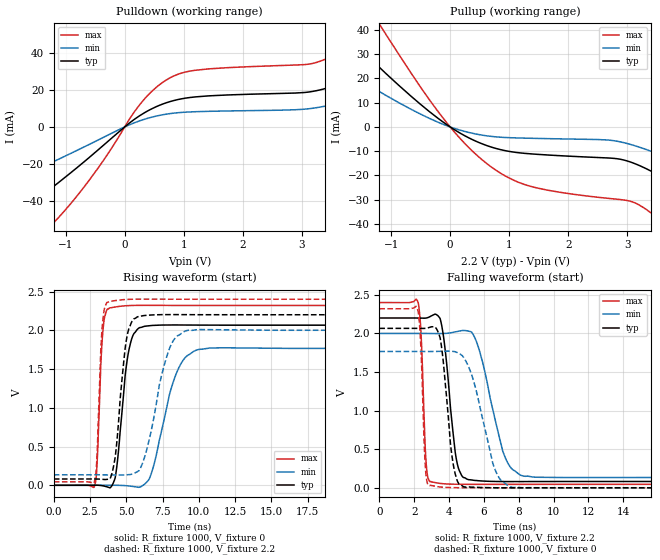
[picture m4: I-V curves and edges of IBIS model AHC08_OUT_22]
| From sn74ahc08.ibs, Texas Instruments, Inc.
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[Model]   AHC08_OUT_22
Model_type  Output
Vref =   0
Rref =   1000
Cref =   50p
Vmeas =   1.1
| variable   typ   min   max
C_comp   3.23pF   2.16pF   4.32pF
| C_pullup   3.15pF   2.16pF   3.84pF
| C_pulldown   3.32pF   2.17pF   4.32pF
[Temperature Range]   40   100   -40
| Ambient temperature   25   85   -40
[Voltage range]   2.2   2   2.4
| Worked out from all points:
|   slope of the pulldown table from 0 to 0.33 V, typ, clamps not added: 43.7 ohm
|   slope of the pullup table from 0 to 0.33 V, typ, clamps not added: 70.6 ohm
|   rising waveform, R_fixture 1000, V_fixture 0: 20-80 % time 645ps typ, 1.37ns min, 302ps max; typ from 0 V to 2.07 V
|   falling waveform, R_fixture 1000, V_fixture 2.2: 20-80 % time 549ps typ, 1.12ns min, 228ps max; typ from 2.2 V to 0.081 V
|   rising waveform, R_fixture 1000, V_fixture 2.2: 20-80 % time 608ps typ, 1.26ns min, 286ps max; typ from 0.081 V to 2.2 V
|   falling waveform, R_fixture 1000, V_fixture 0: 20-80 % time 507ps typ, 1.1ns min, 220ps max; typ from 2.07 V to 0 V
[Pulldown]
| AHC08_OUT_22
|   Voltage   I(typ)   I(min)   I(max)
-5.5V     -129.7mA   -81.96mA   -163.3mA
-3.52V    -85.27mA   -52.66mA   -112.8mA
-2.06V    -52.71mA   -31.41mA   -76.14mA
-1.305V   -34.6mA    -20.22mA   -55.05mA
-620mV    -17.01mA   -9.739mA   -29.56mA
255mV     6.077mA    3.299mA    12.04mA
700mV     12.99mA    6.867mA    25.22mA
3.18V     19.13mA    10.06mA    34.23mA
4.255V    31.65mA    18.76mA    53.81mA
5.495V    55.86mA    35.18mA    90.99mA
6.65V     83.86mA    53.91mA    133.1mA
11V       219.4mA    135.9mA    343.2mA
[Pullup]
| AHC08_OUT_22
|   Voltage   I(typ)   I(min)   I(max)
-5.5V     148.2mA    89.86mA    250.9mA
-2.925V   68.89mA    42.38mA    115.6mA
-1.835V   39.98mA    24.23mA    67.91mA
-1.28V    26.5mA     15.78mA    45.63mA
-75mV     1.249mA    669.7uA    2.265mA
735mV     -8.599mA   -4.003mA   -17.2mA
1.465V    -11.29mA   -4.739mA   -25.17mA
3.09V     -14.81mA   -7.487mA   -30.98mA
3.665V    -21.78mA   -12.51mA   -40.65mA
4.85V     -41.88mA   -25.99mA   -67.56mA
5.975V    -64.03mA   -40.67mA   -94.77mA
11V       -175.9mA   -114.5mA   -224.3mA
[Ramp]
| AHC08_OUT_22
| variable   typ   min   max
dV/dt_r   1.26/7.22E-10   1.08/1.50E-09   1.41/3.33E-10
dV/dt_f   1.30/5.74E-10   1.14/1.16E-09   1.44/2.42E-10
R_load = 1000
[Rising Waveform]
| AHC08_OUT_22
R_fixture =   1000
C_fixture =   0
L_fixture =   0
V_fixture =   0
V_fixture_min = 0
V_fixture_max = 0
|   Time   V(typ)   V(min)   V(max)
0s        158.4pV    433.8pV    54.03pV
2.815ns   921.6uV    339uV      -4.923mV
3.375ns   -6.447mV   471.4uV    1.971V
3.88ns    -33.16mV   455.6uV    2.29V
4.305ns   186.6mV    50.2uV     2.302V
5.19ns    1.758V     -9.166mV   2.318V
6.24ns    2.051V     11.07mV    2.322V
8.45ns    2.068V     1.445V     2.32V
9.995ns   2.067V     1.753V     2.32V
50ns      2.066V     1.766V     2.32V
[Falling Waveform]
| AHC08_OUT_22
R_fixture =   1000
C_fixture =   0
L_fixture =   0
V_fixture =   2.2
V_fixture_min = 2
V_fixture_max = 2.4
|   Time   V(typ)   V(min)   V(max)
0s        2.2V       2V         2.4V
2.24ns    2.199V     2V         2.392V
2.68ns    2.199V     2V         349.2mV
2.915ns   2.218V     1.999V     78.02mV
3.53ns    2.159V     1.998V     55.22mV
4.41ns    387.2mV    2.022V     45.51mV
5.125ns   104.6mV    2.03V      44.03mV
7.16ns    80.3mV     429.3mV    43.92mV
8.28ns    80.22mV    150.6mV    44.1mV
50ns      81.22mV    134.8mV    44.2mV
[Rising Waveform]
| AHC08_OUT_22
R_fixture =   1000
C_fixture =   0
L_fixture =   0
V_fixture =   2.2
V_fixture_min = 2
V_fixture_max = 2.4
|   Time   V(typ)   V(min)   V(max)
0s        81.22mV    134.8mV    44.2mV
2.79ns    81.49mV    135.2mV    41.85mV
2.955ns   81.05mV    135.2mV    296.4mV
3.345ns   76.9mV     134.6mV    2.064V
3.85ns    83.31mV    133.8mV    2.373V
5.025ns   1.899V     135.3mV    2.397V
5.845ns   2.178V     185.1mV    2.401V
7.91ns    2.202V     1.732V     2.401V
9.205ns   2.201V     1.998V     2.4V
50ns      2.2V       2V         2.4V
[Falling Waveform]
| AHC08_OUT_22
R_fixture =   1000
C_fixture =   0
L_fixture =   0
V_fixture =   0
V_fixture_min = 0
V_fixture_max = 0
|   Time   V(typ)   V(min)   V(max)
0s        2.066V     1.766V     2.32V
2.215ns   2.065V     1.766V     2.299V
2.645ns   2.066V     1.766V     266mV
2.88ns    2.078V     1.766V     27.84mV
3.49ns    1.945V     1.768V     9.896mV
4.235ns   315.6mV    1.767V     1.835mV
4.9ns     9.334mV    1.668V     108.2uV
6.595ns   126.8uV    263.8mV    -372.3uV
7.635ns   -669.5uV   4.514mV    -178.8uV
50ns      -2.726nV   -3.941nV   686.7pV
